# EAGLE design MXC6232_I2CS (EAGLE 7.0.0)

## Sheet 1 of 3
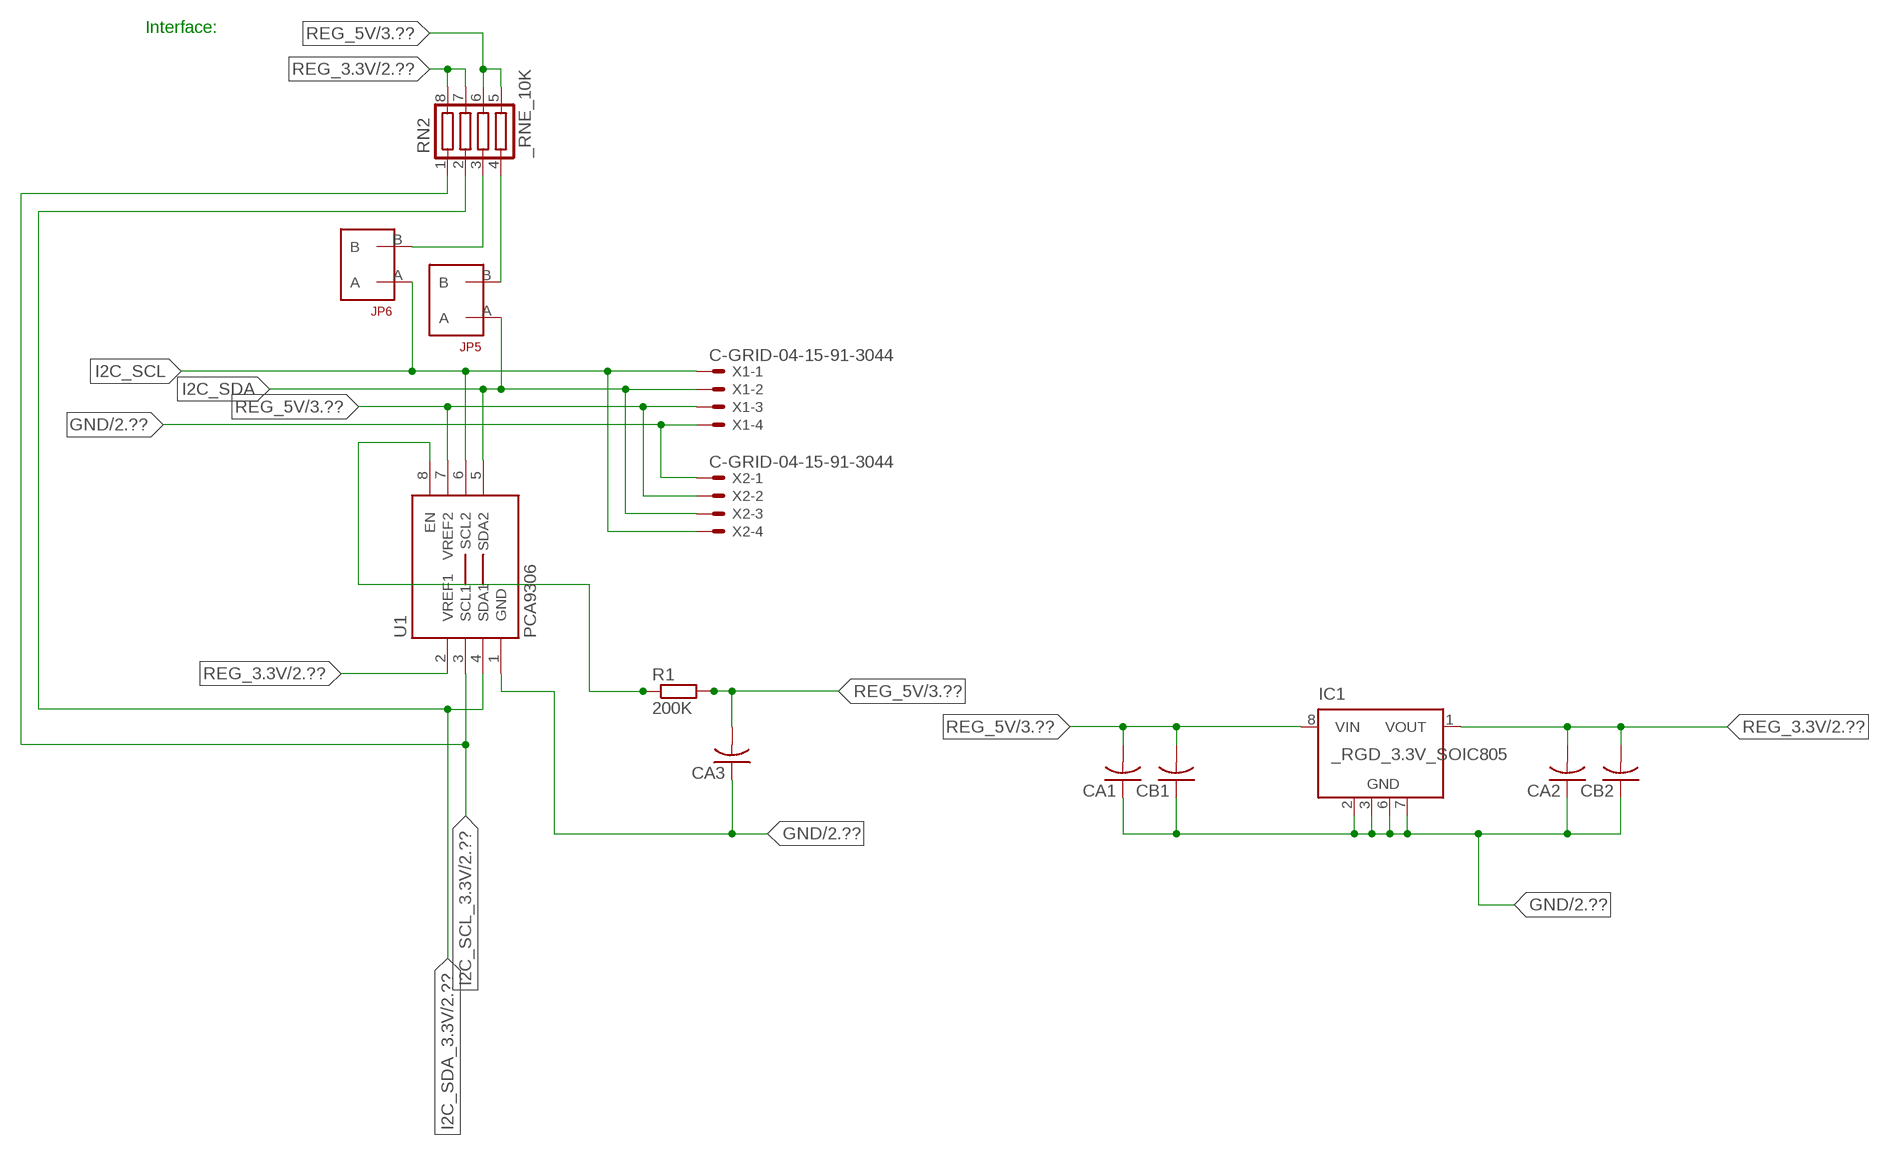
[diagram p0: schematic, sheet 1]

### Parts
CA1  CC1206KRX7R9BB104  [.1UF]
CA2  CC1206KRX7R9BB104  [.1UF]
CA3  CC1206KRX7R9BB104  [.1UF]
CB1  TMK316F106ZL-TC1206K  [TMK316F106ZL-T]
CB2  TMK316F106ZL-TC1206K  [TMK316F106ZL-T]
IC1  _RGD_3.3V_SOIC805  [_RGC_3.3V_SOIC8]
JP5  JUMPER_1X2_2MM  [JUMPER_1X2_2MM]
JP6  JUMPER_1X2_2MM  [JUMPER_1X2_2MM]
R1  200K  RESISTOR_SMT-0603  [R603]
RN2  _RNE_10K  [RNE]
U1  PCA9306  PCA9306_NCD  [PSOP-8]
X1  C-GRID-04-15-91-3044  [15-91-04]
X2  C-GRID-04-15-91-3044  [15-91-04]

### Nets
GND: CA1.1 CA2.1 CA3.1 CB1.1 CB2.1 IC1.2(GND) IC1.3(GND) IC1.6(GND) IC1.7(GND) U1.1(GND) X1.4 X2.1 ; also sheet 2,3
I2C_SCL: JP6.A U1.6(SCL2) X1.1 X2.4
I2C_SCL_3.3V: RN2.1 U1.3(SCL1) ; also sheet 2
I2C_SDA: JP5.A U1.5(SDA2) X1.2 X2.3
I2C_SDA_3.3V: RN2.2 U1.4(SDA1) ; also sheet 2
N$1: JP6.B RN2.3
N$2: JP5.B RN2.4
N$3: R1.1 U1.8(EN)
REG_3.3V: CA2.2 CB2.2 IC1.1(VOUT) RN2.7 RN2.8 U1.2(VREF1) ; also sheet 2
REG_5V: CA1.2 CA3.2 CB1.2 IC1.8(VIN) R1.2 RN2.5 RN2.6 U1.7(VREF2) X1.3 X2.2 ; also sheet 3
Unconnected: IC1.4(NC) IC1.5(NC)

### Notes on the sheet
- Interface:

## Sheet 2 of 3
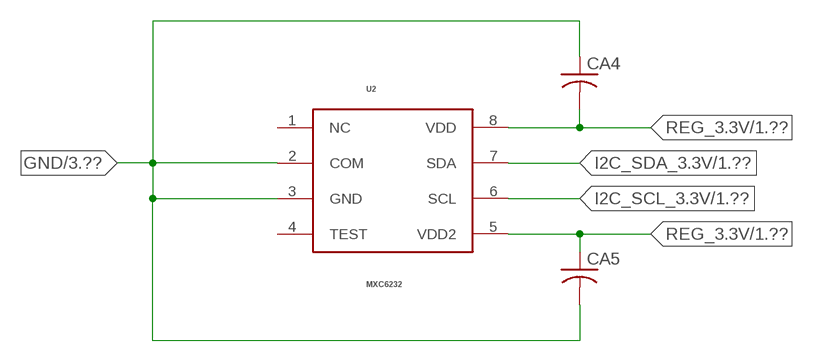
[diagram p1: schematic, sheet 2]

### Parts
CA4  _CA_.10UF_50VC1206K  [_CA_.1UF_50V]
CA5  _CA_.10UF_50VC1206K  [_CA_.1UF_50V]
U2  MXC6232  [MAX6232]

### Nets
GND: CA4.1 CA5.2 U2.2(COM) U2.3(GND) ; also sheet 1,3
I2C_SCL_3.3V: U2.6(SCL) ; also sheet 1
I2C_SDA_3.3V: U2.7(SDA) ; also sheet 1
REG_3.3V: CA4.2 CA5.1 U2.5(VDD2) U2.8(VDD) ; also sheet 1
Unconnected: U2.1(NC) U2.4(TEST)

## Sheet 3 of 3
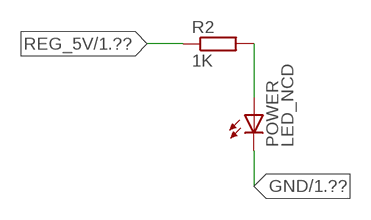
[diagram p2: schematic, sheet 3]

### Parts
POWER  LED_NCD  [CHIPLED_0603]
R2  1K  RESISTOR_SMT-0402  [R402]

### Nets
GND: POWER.C ; also sheet 1,2
N$4: POWER.A R2.2
REG_5V: R2.1 ; also sheet 1

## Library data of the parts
CA1-CA3 = NCD_ULTIMATE_LIBRARY:CC1206KRX7R9BB104: Capacitor CA .1uF 50V SMT C1206K CC1206KRX7R9BB104
CA4 CA5 = NCD_ULTIMATE_LIBRARY:_CA_.10UF_50V: Capacitor .1uF SMT
CB1 CB2 = NCD_ULTIMATE_LIBRARY:TMK316F106ZL-T: Capacitor CB 10uF SMT 1206 TMK316F106ZL-T
IC1 = NCD_ULTIMATE_LIBRARY:_RGD_3.3V_SOIC8: Regulator Linear 3.3V Chip Positive VOLTAGE REGULATOR Digikey 497-1199-2-ND/L78L33ACD13TR
JP5 JP6 = NCD_ULTIMATE_CONNECTORS:JUMPER_1X2_2MM
POWER = NCD_ULTIMATE_LIBRARY:LED_NCD: LED Digikey 754-1132-2-ND/APT2012SRCPRV
R1 R2 = NCD_ULTIMATE_LIBRARY:RESISTOR_SMT: NCD Resistor
RN2 = NCD_ULTIMATE_LIBRARY:_RNE_10K: Resistor Array RNE SMT 10K x 4 Single Resistor Source: http://www.ctscorp.com/components/Datasheets/CTSChipArrayDs.pdf Digikey 742C083103JPTR-ND/742C083103JP; OC_FARNELL: unknown; OC_NEWARK: unknown
U1 = NCD_ULTIMATE_LIBRARY:PCA9306_NCD: NCD Bidirectional I2C level shifter. NOT compatible with all available part number pinout schemes- DOUBLE CHECK!!!; PROD_ID: IC-10023
U2 = NCD_ULTIMATE_bhaskar:MXC6232: http://www.memsic.com/userfiles/files/Datasheets/Accelerometer-Datasheets/MXC6232xMP_Rev_B.pdf
X1 X2 = NCD_ULTIMATE_CONNECTORS:C-GRID-04: CONNECTOR 4-Pos I2C wire to board 2.54 mm (0.100") pitch header Digikey WM1342-ND/0015912045; OC_FARNELL: unknown; OC_NEWARK: unknown

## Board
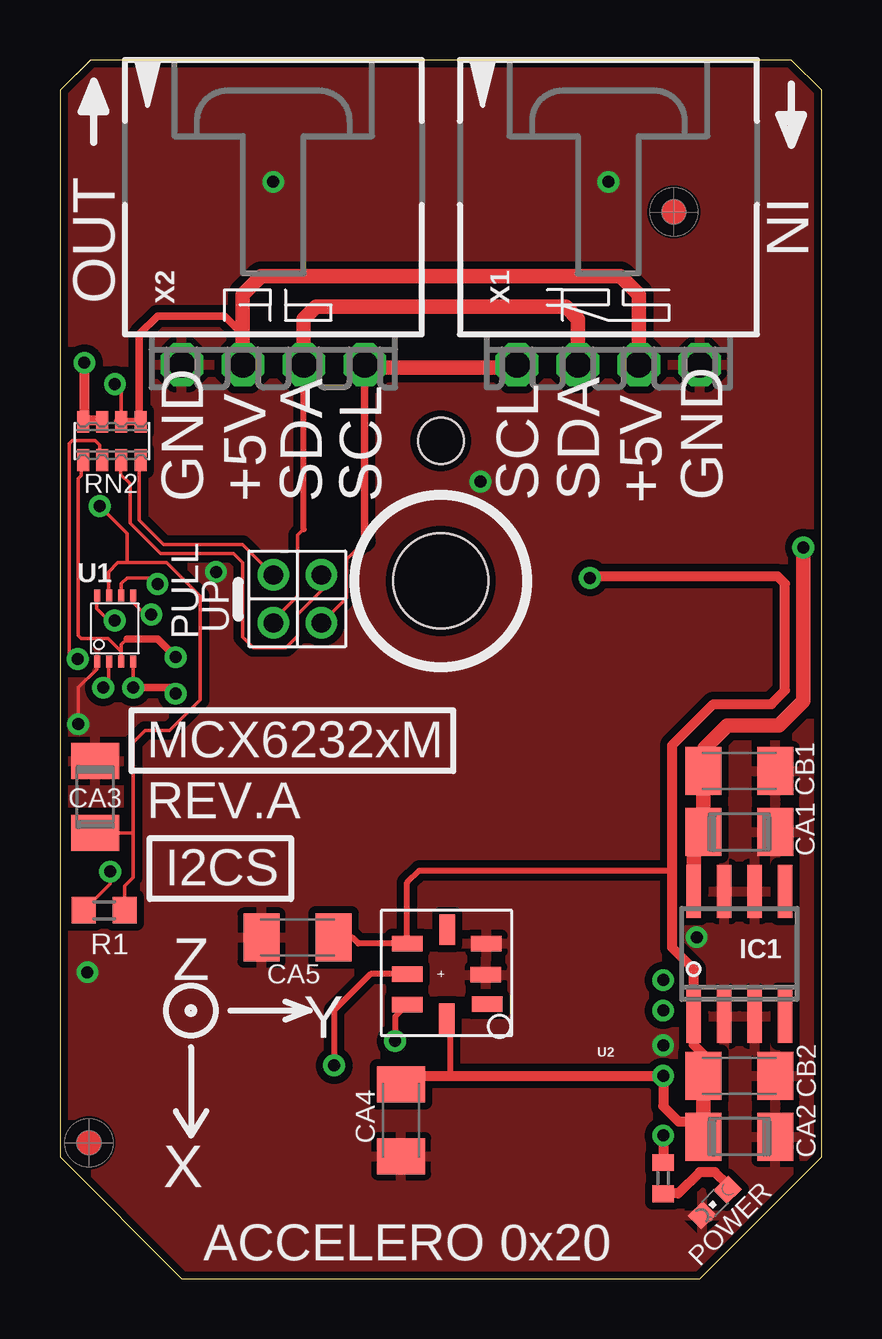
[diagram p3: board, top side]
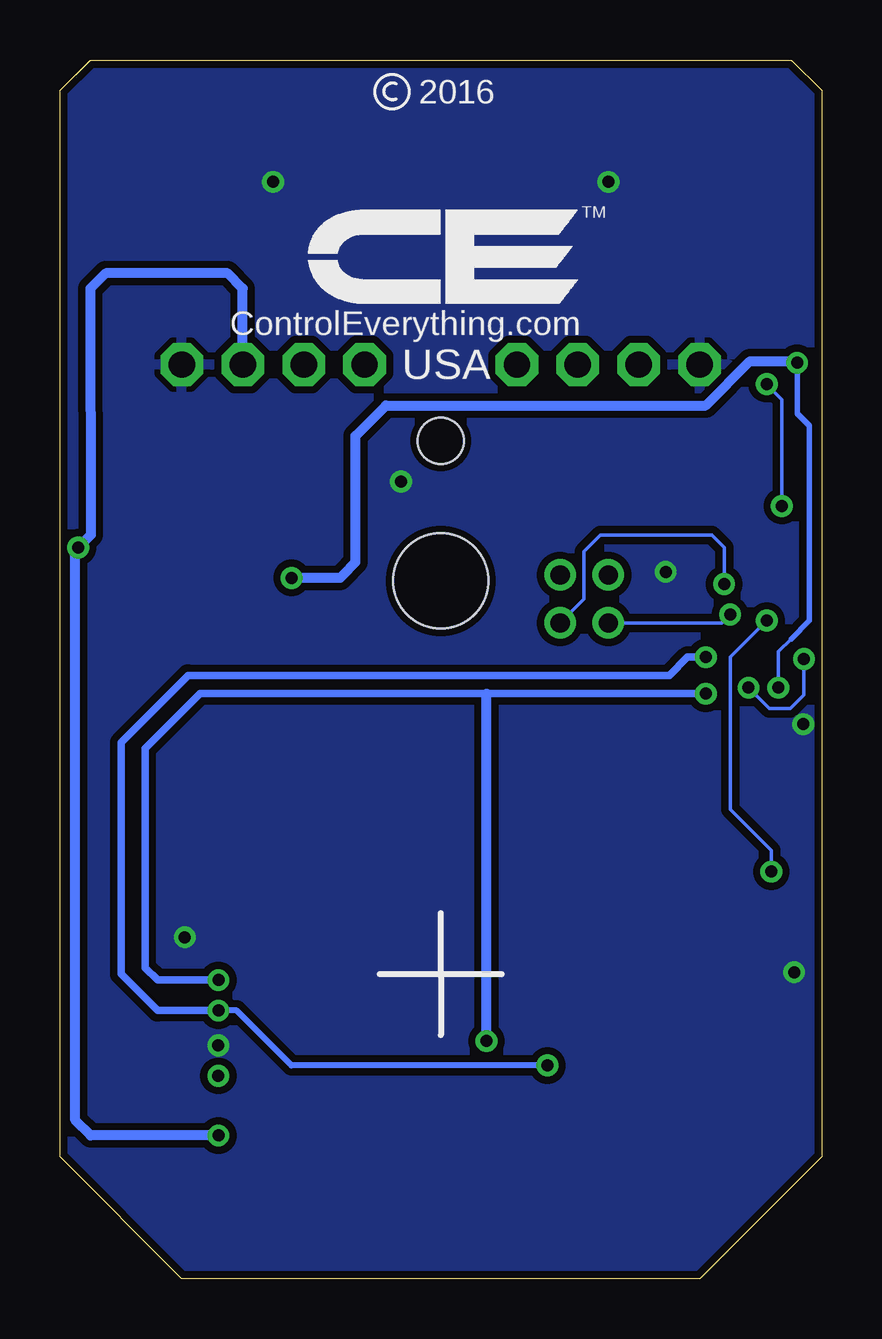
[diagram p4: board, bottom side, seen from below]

Size 31.75 x 50.8 mm. Coordinates in mm from the lower left corner, seen from the top.
Outline: 32 segments
Copper layers (1*16): Top 0.035mm / dielectric 1.5mm / Bottom 0.035mm
Design rules "default": minimum track width 5mil, minimum drill 24mil, track to track 5mil, track to pad 5mil, pad to pad 5mil, via to via 5mil, smd to smd 5mil, copper to edge 10mil, drill to drill 8mil, minimum pad ring 10mil, minimum via ring 8mil, stop-mask expansion 2mil, vias tented up to drill 0mil, thermal gap 10mil
Holes 3.96 mm at 15.88,29.08
Holes 1.91 mm at 15.88,34.93

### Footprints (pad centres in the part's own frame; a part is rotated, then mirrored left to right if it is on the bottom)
.1UF = smd 1.5 x 2: 1 -1.5,0; 2 1.5,0
_CA_.1UF_50V = smd 1.5 x 2: 1 -1.5,0; 2 1.5,0
TMK316F106ZL-T = smd 1.5 x 2: 1 -1.5,0; 2 1.5,0
_RGC_3.3V_SOIC8 = smd 0.6 x 2.2: 1 -1.905,-2.6; 2 -0.635,-2.6; 3 0.635,-2.6; 4 1.905,-2.6; 5 1.905,2.6; 6 0.635,2.6; 7 -0.635,2.6; 8 -1.905,2.6
JUMPER_1X2_2MM = drill 0.8: A 0,2; B 0,0
CHIPLED_0603 = smd 0.8 x 0.876: A 0,-0.75; C 0,0.75
R603 = smd 1 x 1.1: 1 -0.85,0; 2 0.85,0
R402 = smd 0.7 x 0.9: 1 -0.65,0; 2 0.65,0
RNE = smd 0.5 x 0.9: 1 -1.2,-0.8; 2 -0.4,-0.8; 3 0.4,-0.8; 4 1.2,-0.8; 5 1.2,0.8; 6 0.4,0.8; 7 -0.4,0.8; 8 -1.2,0.8
PSOP-8 = smd 0.25 x 0.5: 1 -0.73,-1.37; 2 -0.23,-1.37; 3 0.27,-1.37; 4 0.77,-1.37; 5 0.77,1.38; 6 0.27,1.38; 7 -0.23,1.38; 8 -0.73,1.38
MAX6232 = smd 1.27 x 0.645: 1 -2.06,1.25; 2 -2.01,0.03; 3 -2.03,-1.27; 5 1.27,-1.27; 6 1.27,0; 7 1.27,1.27 | smd 0.645 x 1.27: 4 -0.39,-1.86; 8 -0.38,1.86
15-91-04 = drill 1.1 pad 1.778 octagon: 1 -3.81,-7.62; 2 -1.27,-7.62; 3 1.27,-7.62; 4 3.81,-7.62

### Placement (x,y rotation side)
CA1  28.32,18.62 180 top
CA2  28.32,5.92 180 top
CA3  1.46,20.08 270 top
CA4  14.22,6.6 90 top
CA5  9.91,14.22 180 top
CB1  28.32,21.16 180 top
CB2  28.32,8.46 180 top
IC1  28.32,13.54 0 top
JP5  8.89,29.34 180 top
JP6  10.9,29.34 180 top
POWER  27.3,3.18 135 top
R1  1.84,15.35 0 top
R2  25.15,4.19 270 top
RN2  2.16,34.93 0 top
U1  2.28,27.1 0 top
U2  15.75,12.7 180 top
U$5  [VISION_REF10]  1.21,5.66 90 top
U$28  [VISION_REF10]  25.59,44.46 90 top
X1  22.86,45.72 0 top
X2  8.89,45.72 0 top

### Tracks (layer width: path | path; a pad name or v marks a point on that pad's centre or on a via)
GND  (via drill 0.5)
  Top 0.152: CA3.1 1.52,21.64 1.52,21.59 | U1.1 1.52,25.7 1.52,25.4 0.76,24.64 v0.76,23.11
  other vias: 8.89,45.72 22.86,45.72 25.15,9.73 17.53,33.22 26.55,14.24 1.15,12.78 6.5,29.46
  pour Bottom (isolate 0.305): -0.64,5.08 -0.64,49.53 1.27,51.44 30.48,51.44 32.38,49.53 32.38,5.08 26.67,-0.63 5.08,-0.63
  pour Top (isolate 0.305): 4.45,-1.27 -1.27,4.45 -1.27,50.17 0.64,52.07 31.11,52.07 33.02,50.17 33.02,4.45 27.3,-1.27
I2C_SCL  (via drill 0.5)
  Top 0.152: 12.7,30.73 11.94,29.97 11.94,28.38 JP6.A | v4.06,28.96 3.81,29.21 2.79,29.21 2.55,28.97 U1.6
  Top 0.305: 12.7,30.73 X2.4
  Top 0.406: X2.4 12.7,37.97 | 19.05,37.97 X1.1
  Top 0.61: 12.7,37.97 19.05,37.97
  Bottom 0.152: JP6.A 9.91,28.33 9.91,30.3 9.22,30.99 4.57,30.99 4.06,30.48 v4.06,28.96
I2C_SCL_3.3V  (via drill 0.5)
  Top 0.152: RN2.1 0.89,34.07 0.89,33.48 0.77,33.35 0.77,26.81 0.89,26.68 2.02,26.68 2.55,26.15 U1.3 2.55,26.43 2.79,26.67
  Top 0.254: U2.6 12.95,12.7 11.43,11.18 v11.43,8.89
  Top 0.305: v4.83,25.91 4.06,26.67 2.79,26.67
  Bottom 0.254: v11.43,8.89 22.1,8.89 24.38,11.18 v25.15,11.18
  Bottom 0.305: v25.15,11.18 27.69,11.18 29.21,12.7 29.21,22.35 26.42,25.15 6.35,25.15 5.59,25.91 v4.83,25.91
I2C_SDA  (via drill 0.5)
  Top 0.152: JP5.A 8.89,27.44 9.91,28.45 9.91,30.99 10.16,31.24 | U1.5 3.05,28.19 3.56,27.69 v3.81,27.69
  Top 0.254: 10.16,31.24 10.16,31.25 X2.3
  Top 0.61: X2.3 10.16,40.01 10.67,40.51 21.09,40.51 21.59,40.01 X1.2
  Bottom 0.152: v3.81,27.69 4.16,27.34 JP5.A
I2C_SDA_3.3V  (via drill 0.5)
  Top 0.152: RN2.2 1.65,34.14 1.65,34.75 1.46,34.94 0.51,34.94 0.38,34.81 0.38,25.78 v0.74,25.83 | U1.4 v3.05,24.64
  Top 0.254: U2.7 13.97,10.92 v13.97,9.91
  Top 0.305: v4.83,24.38 4.57,24.64 v3.05,24.64
  Bottom 0.152: v3.05,24.64 2.18,23.77 1.29,23.77 0.74,24.33 v0.74,25.83
  Bottom 0.305: v25.15,12.45 27.69,12.45 28.19,12.95 28.19,22.1 25.91,24.38 13.97,24.38 v4.83,24.38
  Bottom 0.406: v13.97,9.91 13.97,24.38
N$1
  Top 0.152: JP6.B 10.92,29.31 10.92,28.7 9.91,27.69 9.91,26.8 9.42,26.31 8.06,26.31 7.62,26.75 7.62,29.84 7.24,30.23 4.19,30.23 2.92,31.5 2.92,33.15 2.54,33.53 2.54,34.1 RN2.3
  Top 0.305: 2.54,34.02 RN2.3
N$2
  Top 0.152: JP5.B 7.62,30.61 4.32,30.61 3.3,31.62 3.3,34.07 RN2.4
  Top 0.305: 3.37,33.88 RN2.4
N$3  (via drill 0.5)
  Top 0.152: R1.1 2.1,16.46 v2.1,16.97 | U1.8 1.52,28.45 1.52,27.94 2.03,27.43 v2.29,27.43
  Bottom 0.152: v2.29,27.43 3.81,25.91 3.81,19.56 2.1,17.85 v2.1,16.97
N$4
  Top 0.406: POWER.A 27.84,3.92 27.3,4.45 26.67,4.45 25.78,3.56 25.16,3.56 R2.2
REG_3.3V  (via drill 0.5)
  Top 0.152: v1.8,24.64 1.8,24.91 | v1.8,24.64 2.03,24.64 2.03,25.65 2.05,25.68 U1.2 | 1.78,24.64 v1.8,24.64
  Top 0.254: CA5.1 12.19,14.22 12.45,13.97 U2.5 14.48,16.51 14.99,17.02 25.53,17.02 | U2.8 16.26,10.71 16.26,8.46
  Top 0.406: CB2.2 26.82,9.35 26.42,9.75 26.42,10.36 | 26.82,6.55 25.78,6.55 25.15,7.19 v25.15,8.46 16.26,8.46 14.38,8.46 CA4.2 14.45,8.1 14.1,8 14.48,8.26 | IC1.1 26.42,12.9 25.53,13.79 25.53,17.02 25.53,22.24 27.24,23.95 29.66,23.95 30.23,24.52 30.23,28.97 29.91,29.29 22.17,29.29 v22.1,29.21 | 26.52,5.62 CA2.2 | v1.02,38.18 1.02,35.78 | 1.02,35.78 RN2.8 | 1.02,35.78 1.71,35.78 RN2.7
  Top 0.61: CB2.2 26.82,6.55 CA2.2 | 26.42,10.36 IC1.1
  Bottom 0.152: 1.27,26.67 1.8,26.14 v1.8,24.64
  Bottom 0.229: 1.27,26.67 0.51,27.43 0.51,35.56 1.02,36.07 v1.02,38.18
  Bottom 0.406: v1.02,38.18 1.08,38.24 2.99,38.24 4.83,36.4 18.16,36.4 19.43,35.13 19.43,29.87 19.94,29.34 20.07,29.21 v22.1,29.21
REG_5V  (via drill 0.5)
  Top 0.152: RN2.6 2.56,37.01 v2.29,37.29 | 3.05,18.58 3.05,16.73 2.69,16.37 R1.2 | 3.05,18.58 3.05,22.35 3.56,22.86 4.57,22.86 5.84,24.13 5.84,28.45 4.45,29.85 2.79,29.85 | CA3.2 3.05,18.58 | v1.65,32.21 2.79,31.07 2.79,29.85 | 2.79,29.85 2.41,29.85 2.03,29.46 2.03,28.5 U1.7
  Top 0.305: 7.62,39.37 7.5,39.37 | 2.42,35.74 RN2.6 RN2.5 3.31,35.8 3.31,39.37 4.07,40.13 6.86,40.13 7.62,39.37 | X2.2 7.62,39.37
  Top 0.406: v25.15,5.97 R2.1
  Top 0.61: X2.2 7.62,41.02 8.38,41.78 23.37,41.78 24.13,41.02 X1.3 | IC1.8 26.42,18.21 CA1.2 CB1.2 26.86,21.2 26.86,22.11 27.82,23.06 29.98,23.06 30.99,24.08 v30.99,30.48
  Bottom 0.152: v1.65,32.21 1.65,36.65 v2.29,37.29
  Bottom 0.406: X1.3 24.13,41.28 24.77,41.91 29.84,41.91 30.48,41.27 30.47,31 v30.99,30.48 31.11,30.36 31.11,6.6 30.48,5.97 v25.15,5.97

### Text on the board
tNames: IN | OUT | GND | +5V | SDA | SCL | SCL | SDA | +5V | GND | PULL | UP | MCX6232xM | REV.A | I2CS | Z | Y | X | ACCELERO 0x20
bNames: 2016 | TM | ControlEverything.com | USA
